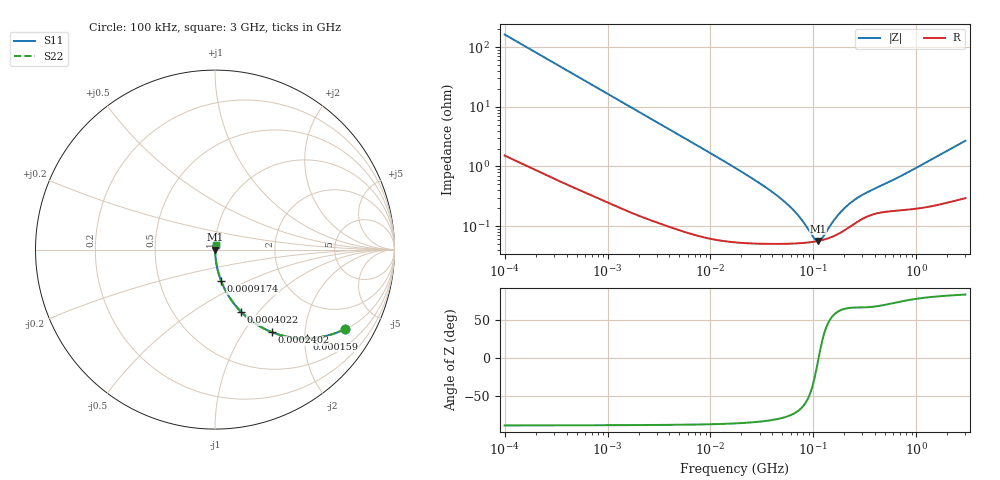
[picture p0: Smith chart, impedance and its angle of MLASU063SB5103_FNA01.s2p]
! MLASU063SB5103_FNA01  S-PARAMETER MODEL  ( Standard Model )
! Model Generated by TAIYO YUDEN Corporation (http://www.ty-top.com)
! Version 1.0
! TAIYO YUDEN Control No. 220601
! Copyright(c) 2013 TAIYO YUDEN CO.,LTD. All Rights Reserved.
! Product Description (link to TY-COMPAS)
! https://ds.yuden.co.jp/TYCOMPAS/or/detail?pn=MLASU063SB5103KFNA01&u=M
! Products Name : Multilayer Ceramic Capacitors
! Characteristics :
!  Capacitance : 0.01 [uF] , Rated Voltage : 50 [V] , TCC : B / X5R
!  Case Size : 0.6 x 0.3 / 0.024 x 0.012 [mm/inch] , Thickness : 0.3 / 0.012 [mm/inch]
!  (Conditions: Temperature = 25 [degC] , DC Bias Voltage = 0 [V])
! External Node Assignments :
!  1  o---| |---o  2
! GND o---------o GND
! Frequency Range : 100kHz  -  3GHz  [ 401 STEP ]
# MHZ S RI R 50
! Freq[MHz].  S11 Real  S11 Imag  S21 Real  S21 Imag  S12 Real  S12 Imag  S22 Real  S22 Imag
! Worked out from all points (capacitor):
!   401 points, 100 kHz to 3 GHz, reference 50 ohm
!   read as one part in series: C = 9.78 nF near 105.3 kHz
!   lowest |Z| = 56.7 mohm at 110.8 MHz (marker M1)
!   series resonance near 112.5 MHz, so ESL is about 200 pH
!   S11 on the Smith chart (normalised r, x): 100 kHz: 1.03, -3.25; 159 kHz: 1.02, -2.05; 240.2 kHz: 1.02, -1.36; 402.2 kHz: 1.01, -0.82; 917.4 kHz: 1.01, -0.36; 3 GHz: 1.01, +0.05
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0.1  0.7236 -0.4425  0.2764 0.4425  0.2764 0.4425  0.7236 -0.4425
0.159027  0.5122 -0.4947  0.4878 0.4947  0.4878 0.4947  0.5122 -0.4947
0.24019  0.3183 -0.4603  0.6817 0.4603  0.6817 0.4603  0.3183 -0.4603
0.402172  0.1456 -0.3466  0.8544 0.3466  0.8544 0.3466  0.1456 -0.3466
0.562235  0.0817 -0.2674  0.9183 0.2674  0.9183 0.2674  0.0817 -0.2674
0.917447  0.0338 -0.1733  0.9662 0.1733  0.9662 0.1733  0.0338 -0.1733
1.61742  0.0121 -0.1011  0.9879 0.1011  0.9879 0.1011  0.0121 -0.1011
3.161081  0.00388 -0.0525  0.9961 0.0525  0.9961 0.0525  0.00388 -0.0525
17.7727  0.000619 -0.00925  0.9994 0.00925  0.9994 0.00925  0.000619 -0.00925
34.73492  0.000525 -0.0044  0.9995 0.0044  0.9995 0.0044  0.000525 -0.0044
53.83243  0.000513 -0.00242  0.9995 0.00242  0.9995 0.00242  0.000513 -0.00242
73.34282  0.00052 -0.00133  0.9995 0.00133  0.9995 0.00133  0.00052 -0.00133
97.38194  0.000544 -0.000439  0.9995 0.000439  0.9995 0.000439  0.000544 -0.000439
105.21  0.000555 -0.000203  0.9994 0.000203  0.9994 0.000203  0.000555 -0.000203
110.7752  0.000564 -4.7e-05  0.9994 4.7e-05  0.9994 4.7e-05  0.000564 -4.7e-05
116.6348  0.000575 0.000109  0.9994 -0.000109  0.9994 -0.000109  0.000575 0.000109
122.8043  0.000588 0.000266  0.9994 -0.000266  0.9994 -0.000266  0.000588 0.000266
167.3121  0.000717 0.00123  0.9993 -0.00123  0.9993 -0.00123  0.000717 0.00123
227.9507  0.000991 0.00223  0.999 -0.00223  0.999 -0.00223  0.000991 0.00223
310.5665  0.00138 0.00318  0.9986 -0.00318  0.9986 -0.00318  0.00138 0.00318
547.5153  0.0018 0.00523  0.9982 -0.00523  0.9982 -0.00523  0.0018 0.00523
3000  0.00365 0.0266  0.9963 -0.0266  0.9963 -0.0266  0.00365 0.0266
